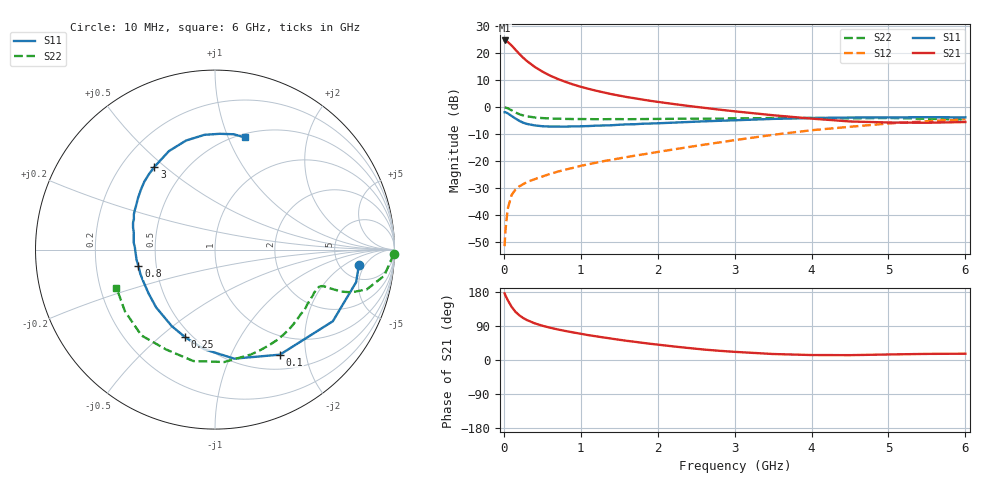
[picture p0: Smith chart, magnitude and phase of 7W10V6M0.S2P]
! Infineon Technologies  Discrete & RF Semiconductors
! BFS17W
! Si NPN RF Bipolar Junction Transistor in SOT323
! VCE = 10 V  IC = 6 mA
! Common Emitter S-Parameters:  August  1999
# GHz  S  MA  R  50
!  f  S11  S21  S12  S22
! GHz  MAG  ANG  MAG  ANG  MAG  ANG  MAG  ANG
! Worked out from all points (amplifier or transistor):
!   36 points, 10 MHz to 6 GHz, reference 50 ohm
!   highest |S21| = 24.6 dB at 10 MHz (marker M1)
!   |S21| within 3 dB of that: start of sweep to 137.4 MHz
!   unconditionally stable (mu >= 1): 552 MHz to 2.247 GHz; 5.396 GHz to end of sweep
!   at 250 MHz: K = 0.63, MSG = 23.4 dB, |S12| = -28.5 dB
!   at 1.4 GHz: K = 1.18, MAG = 9.5 dB, |S12| = -19.5 dB
!   at 6 GHz: K = 1.04, MAG = -1.8 dB, |S12| = -4.5 dB
!   S11 on the Smith chart (normalised r, x): 10 MHz: 7.40, -3.74; 100 MHz: 0.70, -1.56; 250 MHz: 0.46, -0.61; 800 MHz: 0.40, -0.09; 3 GHz: 0.34, +0.46; 6 GHz: 0.53, +1.15
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0.01  0.8062 -6.3  17.03 175.7  0.0027 77.9  0.9951 -1.4
0.02  0.807 -13.0  16.87 170.8  0.0051 88.0  0.981 -3.7
0.05  0.7683 -31.3  16.03 158.1  0.0131 79.3  0.9538 -8.8
0.1  0.688 -58.3  13.8 140.7  0.0237 64.1  0.874 -14.7
0.15  0.6169 -80.0  11.52 127.4  0.0299 57.1  0.7961 -17.4
0.2  0.5587 -96.1  9.677 118.1  0.0343 55.2  0.7415 -18.4
0.25  0.5161 -108.7  8.203 111.0  0.0376 52.3  0.7018 -18.5
0.3  0.4896 -119.5  7.099 105.4  0.0413 52.0  0.6773 -18.6
0.4  0.4597 -135.5  5.549 96.9  0.0466 53.4  0.6439 -18.6
0.5  0.4436 -146.4  4.536 90.5  0.0522 55.7  0.6276 -18.9
0.6  0.4372 -155.0  3.823 85.3  0.0583 57.8  0.6166 -19.6
0.8  0.4365 -168.0  2.93 76.6  0.0701 60.4  0.6057 -22.1
0.9  0.4408 -172.6  2.621 72.8  0.0754 62.0  0.6021 -23.6
1.1  0.4467 178.4  2.177 65.6  0.0881 64.1  0.5998 -26.9
1.4  0.4623 168.1  1.736 56.4  0.1063 66.9  0.6003 -32.7
1.6  0.4805 161.9  1.535 50.6  0.1195 68.1  0.5981 -36.9
2.2  0.5165 146.1  1.144 35.9  0.1648 71.9  0.6083 -50.9
3  0.5712 126.3  0.836 21.5  0.2451 71.8  0.6176 -71.1
3.5  0.6058 115.1  0.708 15.8  0.308 69.1  0.6286 -85.2
4.5  0.6421 95.3  0.543 12.8  0.4332 57.6  0.6196 -116.0
5.5  0.651 80.8  0.514 16.1  0.5491 44.2  0.6082 -145.6
6  0.6468 75.2  0.53 16.6  0.5944 37.5  0.5888 -158.8
